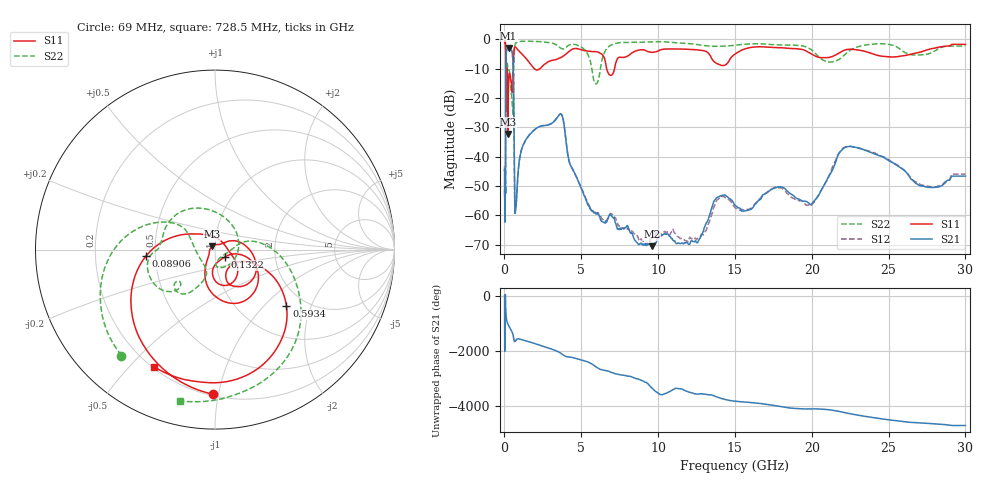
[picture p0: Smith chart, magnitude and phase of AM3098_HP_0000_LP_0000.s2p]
! Date/Time: Thu, Feb 28, 2019 8:30 AM
! Network Analyzer: Agilent Technologies E8364B Rev: A.07.50.67
! Sweep from 0.010 to 30.000 GHz, 1601 Points, Sweep Type: LOG
! Power Supply: 5.022 V, 0.002 A
# Hz S DB R 50
!freq MagS11 AngS11 MagS21 AngS21 MagS12 AngS12 MagS22 AngS22
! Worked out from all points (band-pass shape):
!   1601 points, 10 MHz to 30 GHz, reference 50 ohm
!   highest |S21| = -2.95 dB at 266.5 MHz (marker M1); lowest = -70.5 dB at 9.586 GHz (marker M2)
!   |S21| within 3 dB of the highest: 103.6 MHz to 533.9 MHz (430.3 MHz wide, 135 % of centre)
!   lowest |S11| = -32.2 dB at 227 MHz (marker M3), VSWR 1.05, Z = 48.4 + j1.76 ohm
!   |S11| at or under -10 dB: 175.7 MHz to 562 MHz (386.3 MHz wide, 105 % of centre); 1.951 GHz to 2.283 GHz (332.1 MHz wide, 15.7 % of centre); 6.652 GHz to 7.164 GHz (511.8 MHz wide, 7.41 % of centre)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
!   |S22| runs from -25.5 to -0.5 dB; largest |S21 - S12| = 0.013
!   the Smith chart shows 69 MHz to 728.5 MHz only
!   S11 on the Smith chart (normalised r, x): 69 MHz: 0.21, -0.97; 89.06 MHz: 0.44, -0.04; 132.2 MHz: 1.11, -0.09; 593.4 MHz: 1.61, -1.36; 728.5 MHz: 0.21, -0.59
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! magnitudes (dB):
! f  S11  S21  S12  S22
! 10 MHz  -0.4  -44.7  -43.2  -0.5
! 38.04 MHz  -0.5  -61.3  -60.0  -0.8
! 69 MHz  -1.9  -51.3  -50.9  -2.1
! 89.06 MHz  -8.3  -18.3  -18.2  -10.1
! 97.94 MHz  -24.6  -7.7  -7.7  -18.2
! 132.2 MHz  -23.2  -3.7  -3.7  -11.5
! 144.7 MHz  -13.3  -3.5  -3.4  -10.1
! 188.7 MHz  -11.8  -3.3  -3.3  -8.4
! 227 MHz  -32.2  -3.0  -3.0  -10.0
! 266.5 MHz  -15.1  -2.9  -2.9  -10.5
! 550.5 MHz  -11.9  -7.2  -7.2  -25.3
! 593.4 MHz  -5.9  -15.9  -15.8  -11.8
! 665.8 MHz  -2.6  -55.2  -54.2  -2.3
! 728.5 MHz  -2.7  -58.0  -56.9  -1.3
! 2.084 GHz  -10.4  -30.3  -30.3  -0.7
! 3.686 GHz  -6.1  -25.5  -25.5  -3.1
! 5.959 GHz  -4.2  -59.6  -59.1  -15.2
! 7.926 GHz  -5.9  -64.0  -64.8  -1.0
! 9.586 GHz  -4.4  -70.5  -67.8  -0.8
! 19.8 GHz  -4.4  -55.8  -56.4  -3.0
! 22.67 GHz  -3.4  -36.6  -36.7  -3.2
! 30 GHz  -1.7  -46.6  -46.0  -2.3
